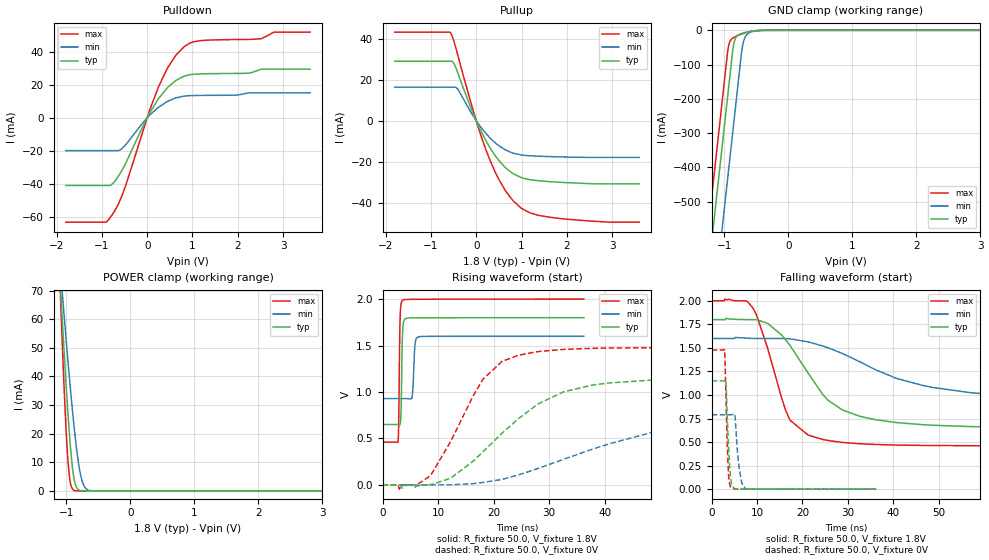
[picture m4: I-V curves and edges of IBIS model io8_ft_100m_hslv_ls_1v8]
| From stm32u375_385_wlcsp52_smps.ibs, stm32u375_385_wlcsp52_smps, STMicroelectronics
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[Model]   io8_ft_100m_hslv_ls_1v8
Model_type I/O
Polarity   Non-Inverting
Enable   Active-Low
| CAP_THRESHOLD on pad IOFT is "UDTCAPC" :
| Rising=30.0% of vddiom   Falling=70.0% of vddiom
| C_comp min and max val. don't necessarily correlate with the min and max pvt
| but are the smallest and greatest pad capacitance found.
| var   typ   min   max
C_comp   3.41781pF  3.41646pF  3.48186pF
|C_comp_pullup   1.92518pF  1.84292pF  2.10196pF
|C_comp_pulldown   1.49264pF  1.57354pF  1.37990pF
Vinl = 800.0mV
Vinh = 1.0V
Vmeas = 900.0mV   | Reference voltage for timing measurements
Cref  = 50.0pF   | Timing specification test load capacitance value
Rref  = 1.0MOhm   | Timing specification test load resistance value
Vref  = 990.0mV   | Timing specification test load voltage
[Model Spec]
| TIME_THRESHOLD on pin ZIV11 is "CMOS" :
| Rising=50.0% of vdd   Falling=50.0% of vdd
Vinl 694.50000mV 619.50000mV 778.50000mV
Vinh 1.08350V 957.50000mV 1.18750V
| variable   typ   min   max
[Temperature Range] 25.0 130.0 -40.0
| variable   typ   min   max
[Voltage Range] 1.8V 1.6V 2.0V
| variable   typ   min   max
[POWER Clamp Reference] 1.8V 1.6V 2.0V
| variable   typ   min   max
[GND Clamp Reference] 0V 0V 0V
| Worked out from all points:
|   slope of the pulldown table from 0 to 0.27 V, typ, clamps not added: 21.9 ohm
|   slope of the pullup table from 0 to 0.27 V, typ, clamps not added: 22.7 ohm
|   GND clamp passes 1 mA (typ) near -0.50 V on its own axis
|   POWER clamp passes 1 mA (typ) near -0.83 V on its own axis
|   rising waveform, R_fixture 50.0, V_fixture 1.8V: 20-80 % time 201ps typ, 297ps min, 190ps max; typ from 0.65 V to 1.8 V
|   falling waveform, R_fixture 50.0, V_fixture 1.8V: 20-80 % time 11ns typ, 23.8ns min, 5.96ns max; typ from 1.8 V to 0.65 V
|   rising waveform, R_fixture 50.0, V_fixture 0V: 20-80 % time 14ns typ, 27.3ns min, 8.31ns max; typ from 0 V to 1.15 V
|   falling waveform, R_fixture 50.0, V_fixture 0V: 20-80 % time 680ps typ, 935ps min, 543ps max; typ from 1.15 V to 0 V
[POWER Clamp]
-1.8V     399.1mA    292.1mA    557.7mA
-1.09V    71.2mA     76.8mA     67.14mA
-1.08V    67.05mA    73.98mA    61.2mA
-1.06V    58.89mA    68.38mA    49.67mA
-1.02V    43.22mA    57.4mA     28.67mA
-980mV    28.81mA    46.77mA    12.28mA
-940mV    16.45mA    36.61mA    3.257mA
-880mV    4.35mA     22.67mA    225.4uA
-820mV    610.4uA    11.29mA    13uA
-770mV    97.5uA     4.87mA     1.193uA
-640mV    753.9nA    196uA      2.492nA
3.6V      0A         0A         0A
[GND Clamp]
-1.8V     -1.64A     -1.88A     -1.509A
-1.24V    -688.2mA   -927.9mA   -557mA
-1.05V    -365.2mA   -604.9mA   -234mA
-950mV    -195.2mA   -434.9mA   -64mA
-930mV    -161.2mA   -400.9mA   -41.59mA
-870mV    -59.19mA   -298.9mA   -22.94mA
-850mV    -36.73mA   -264.9mA   -20.65mA
-770mV    -12.21mA   -128.9mA   -13.73mA
-730mV    -9.139mA   -62.1mA    -10.81mA
-690mV    -6.97mA    -26.33mA   -8.198mA
-530mV    -1.564mA   -2.413mA   -1.407mA
3.6V      1.228nA    159.5nA    526.9pA
| variable   typ   min   max
[Pullup Reference] 1.8V 1.6V 2.0V
| variable   typ   min   max
[Pulldown Reference] 0V 0V 0V
[Pullup]
-1.8V     29.01mA    16.34mA    43.22mA
-570mV    29.01mA    16.34mA    42.9mA
-500mV    28.15mA    16.34mA    39.2mA
-410mV    23.5mA     15.42mA    32.16mA
10mV      -503.1uA   -323.9uA   -726uA
290mV     -12.65mA   -8.055mA   -18.46mA
630mV     -22.57mA   -14.06mA   -33.59mA
810mV     -25.79mA   -15.81mA   -38.95mA
1V        -27.82mA   -16.74mA   -42.77mA
1.37V     -29.26mA   -17.3mA    -46.1mA
1.74V     -29.87mA   -17.56mA   -47.39mA
3.6V      -30.8mA    -17.88mA   -49.48mA
[Pulldown]
-1.8V     -41.16mA   -19.96mA   -63.43mA
-920mV    -41.16mA   -19.96mA   -63.43mA
-780mV    -40.43mA   -19.96mA   -59.18mA
-510mV    -29.46mA   -17.38mA   -43.8mA
0V        0A         -390fA     0A
250mV     11.64mA    6.428mA    18.87mA
460mV     18.67mA    10.12mA    30.76mA
810mV     25.21mA    13.14mA    43.03mA
1.18V     26.67mA    13.59mA    46.9mA
2.5V      29.31mA    15.12mA    47.95mA
2.81V     29.55mA    15.12mA    52.03mA
3.6V      29.55mA    15.12mA    52.05mA
[Ramp]
dV/dt_r 690.02014mV/13.59272ns 474.31692mV/26.95383ns 886.36616mV/7.8629ns
dV/dt_f 689.75416mV/10.78748ns 402.9603mV/23.28692ns 923.68048mV/5.78655ns
R_load = 50.0
| Removed startup time: 0s 0s 0s  .
| Removed end time: 36.25ns.
[Rising Waveform]
R_fixture   = 50.0
V_fixture   = 1.8V
V_fixture_min = 1.6V
V_fixture_max = 2.0V
0s        650.4mV    928.4mV    460.5mV
2.8ns     650.4mV    928.4mV    474.2mV
2.9ns     650.4mV    928.4mV    630.1mV
3.15ns    650mV      928.4mV    1.772V
3.35ns    835.1mV    928.4mV    1.952V
3.6ns     1.629V     928.4mV    1.988V
5.3ns     1.798V     940.3mV    1.997V
5.85ns    1.798V     1.513V     1.998V
6.65ns    1.798V     1.596V     1.998V
36.25ns   1.8V       1.6V       2V
| Removed startup time: 0s 0s 0s  .
| Removed end time: 399.25ns.
[Falling Waveform]
R_fixture   = 50.0
V_fixture   = 1.8V
V_fixture_min = 1.6V
V_fixture_max = 2.0V
0s        1.8V       1.6V       2V
8.15ns    1.8V       1.602V     1.979V
9.95ns    1.8V       1.6V       1.842V
12.35ns   1.76V      1.6V       1.496V
17.3ns    1.524V     1.596V     730.8mV
24.45ns   1.008V     1.521V     528.1mV
28.85ns   840.2mV    1.44V      496.2mV
48.9ns    678.3mV    1.078V     463.4mV
81.5ns    652.5mV    956.5mV    460.6mV
399.3ns   650.4mV    928.4mV    460.5mV
| Removed startup time: 0s 0s 0s  .
| Removed end time: 399.2ns.
[Rising Waveform]
R_fixture   = 50.0
V_fixture   = 0V
V_fixture_min = 0V
V_fixture_max = 0V
0s        4.611nV    97.7nV     3.397nV
3.05ns    -519uV     -113.7nV   -46.12mV
8.85ns    5.134mV    -364.5uV   120.8mV
12.2ns    69.91mV    426.9uV    461.2mV
18.05ns   354.9mV    26.1mV     1.135V
21.5ns    556.1mV    58.73mV    1.329V
32.6ns    1.002V     276.1mV    1.458V
57.05ns   1.142V     661.1mV    1.477V
81.5ns    1.149V     765.3mV    1.477V
399.2ns   1.15V      790.5mV    1.477V
| Removed startup time: 0s 0s 0s  .
| Removed end time: 36.25ns.
[Falling Waveform]
R_fixture   = 50.0
V_fixture   = 0V
V_fixture_min = 0V
V_fixture_max = 0V
0s        1.15V      790.6mV    1.477V
2.85ns    1.15V      790.6mV    1.483V
3.15ns    1.14V      790.6mV    1.004V
3.65ns    538.2mV    790.6mV    239mV
3.95ns    275.7mV    790.6mV    65.07mV
4.4ns     55.88mV    790.7mV    11.52mV
5.1ns     5.647mV    795.1mV    2.629mV
6.15ns    1.434mV    200.1mV    1.766mV
7.4ns     1.055mV    6.751mV    1.677mV
36.25ns   86.44uV    189.5uV    34.21uV
